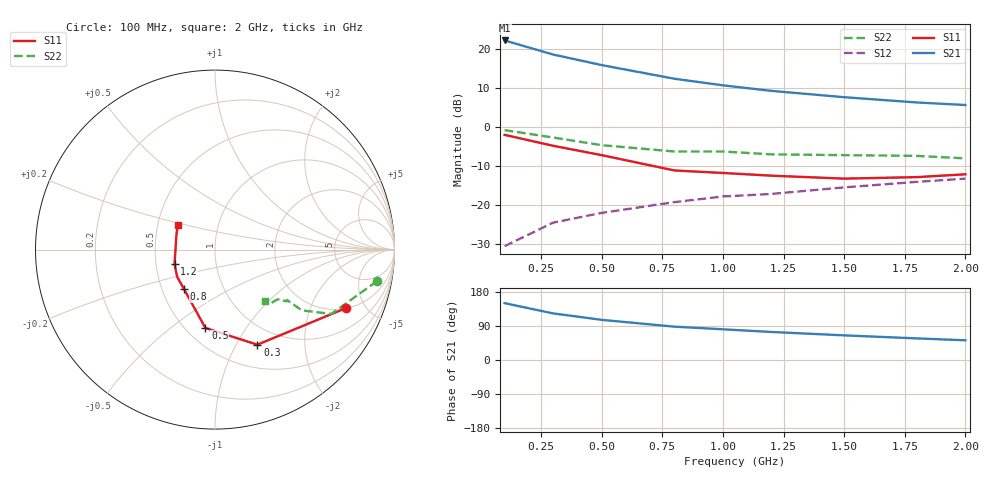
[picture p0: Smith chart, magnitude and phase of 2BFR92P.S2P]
!BFR92P,Si-NPN-RF Transistor in SOT 23-package
!Vce = 6 V, Ic = 5 mA
# GHZ S MA R 50
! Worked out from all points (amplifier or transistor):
!   9 points, 100 MHz to 2 GHz, reference 50 ohm
!   highest |S21| = 22.3 dB at 100 MHz (marker M1)
!   |S21| within 3 dB of that: start of sweep to 266.5 MHz
!   unconditionally stable (mu >= 1): 1.15 GHz to end of sweep
!   at 300 MHz: K = 0.48, MSG = 21.5 dB, |S12| = -24.4 dB
!   at 1 GHz: K = 0.92, MSG = 14.2 dB, |S12| = -17.7 dB
!   at 2 GHz: K = 1.04, MAG = 8.2 dB, |S12| = -13.2 dB
!   S11 on the Smith chart (normalised r, x): 100 MHz: 2.02, -3.65; 300 MHz: 0.77, -1.23; 500 MHz: 0.62, -0.67; 800 MHz: 0.65, -0.31; 1.2 GHz: 0.62, -0.11; 2 GHz: 0.63, +0.19
0.1  0.8 -24.0  12.96 150.0  0.03 75.0  0.92 -11.0
0.3  0.58 -66.0  8.56 123.0  0.06 61.0  0.74 -29.0
0.5  0.44 -97.0  6.27 106.0  0.08 58.0  0.59 -35.0
0.8  0.28 -128.0  4.19 88.0  0.11 57.0  0.49 -35.0
1  0.26 -144.0  3.45 81.0  0.13 59.0  0.49 -36.0
1.2  0.24 -160.0  2.93 74.0  0.14 58.0  0.45 -38.0
1.5  0.22 179.0  2.43 65.0  0.17 59.0  0.44 -40.0
1.8  0.23 159.0  2.08 57.0  0.2 59.0  0.43 -45.0
2  0.25 146.0  1.93 52.0  0.22 58.0  0.4 -46.0
